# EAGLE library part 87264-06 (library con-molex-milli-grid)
RECEPTACAL
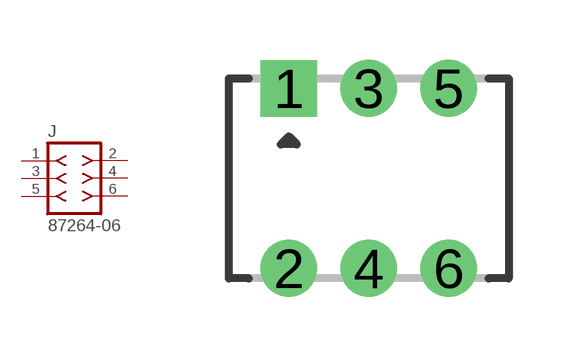
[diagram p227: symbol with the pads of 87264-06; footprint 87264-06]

Designator prefix J

## 87264-06  [87264-06]
1  1  pas
2  2  pas
3  3  pas
4  4  pas
5  5  pas
6  6  pas

## Footprint 87264-06 (pad centres in mm)
RECEPTACAL Dual Row, Side Entry
drill 0.914 square: 1 -2,2.25
drill 0.914: 2 -2,-2.25; 3 0,2.25; 4 0,-2.25; 5 2,2.25; 6 2,-2.25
